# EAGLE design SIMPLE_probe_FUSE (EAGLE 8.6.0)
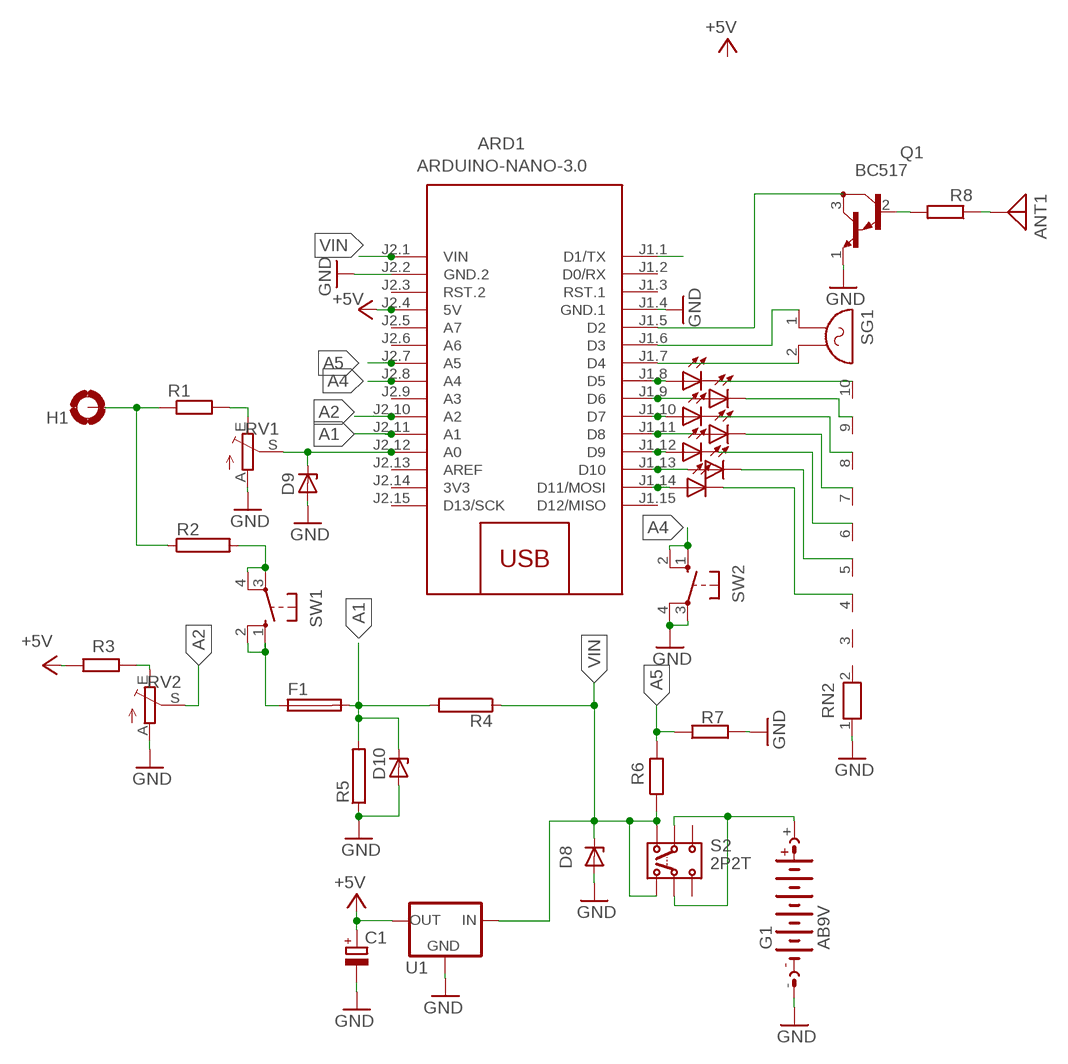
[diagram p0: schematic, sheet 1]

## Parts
ANT1  ANTENNA  [PAD-01]
ARD1  ARDUINO-NANO-3.0  [ARDUINO-NANO-3.0]
C1  CPOL-EUE2.5-6  [E2,5-6]
D1  LED5MM  [LED5MM]
D2  LED5MM  [LED5MM]
D3  LED5MM  [LED5MM]
D4  LED5MM  [LED5MM]
D5  LED5MM  [LED5MM]
D6  LED5MM  [LED5MM]
D7  LED5MM  [LED5MM]
D8  BZY97  [F126Z12]
D9  BZY97  [F126Z12]
D10  BZY97  [F126Z12]
F1  TE5  [TE5]
G1  AB9V  [AB9V]
H1  MOUNT-PAD-ROUND5.0  [5,0-PAD]
Q1  BC517  [TO92]
R1  R-EU_0617/22  [0617/22]
R2  RRWM4X22  [RWM4X22]
R3  R-EU_R1206  [R1206]
R4  RRWM4X22  [RWM4X22]
R5  RRWM4X22  [RWM4X22]
R6  R-EU_R1206  [R1206]
R7  R-EU_R1206  [R1206]
R8  R-EU_R1206  [R1206]
RN2  RN09  [RN-10]
RV1  TRIM_EU-CT6  [CT6]
RV2  TRIM_EU-CT6  [CT6]
S2  2P2T  [2P2T]
SG1  F/HGP  [F/HGP]
SW1  40-XX  [B3F-40XX]
SW2  40-XX  [B3F-40XX]
U1  78LXX  [78LXX]

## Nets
+5V: ARD1.J2.4(5V) C1.+ R3.1 U1.OUT
A1: ARD1.J2.11(A1) D10.C F1.2 R4.2 R5.2
A2: ARD1.J2.10(A2) RV2.S
A4: ARD1.J2.8(A4) SW2.1(S) SW2.2(S1)
A5: ARD1.J2.7(A5) R6.2 R7.1
GND: ARD1.J1.4(GND.1) ARD1.J2.2(GND.2) C1.- D8.A D9.A D10.A G1.- Q1.1(E) R5.1 R7.2 RN2.1 RV1.A RV2.A SW2.3(P) SW2.4(P1) U1.GND
N$1: ARD1.J1.1(D1/TX)
N$2: Q1.2(B) R8.2
N$3: ANT1.1 R8.1
N$4: R1.2 RV1.E
N$5: ARD1.J1.8(D5) D6.A
N$6: D6.K(C) RN2.10
N$7: ARD1.J1.9(D6) D3.A
N$8: D3.K(C) RN2.9
N$9: ARD1.J1.10(D7) D5.A
N$10: ARD1.J1.11(D8) D1.A
N$11: ARD1.J1.12(D9) D2.A
N$12: ARD1.J1.13(D10) D4.A
N$13: ARD1.J1.14(D11/MOSI) D7.A
N$14: D5.K(C) RN2.8
N$15: D1.K(C) RN2.7
N$16: D2.K(C) RN2.6
N$17: ARD1.J1.7(D4) SG1.2
N$18: ARD1.J1.6(D3) SG1.1
N$19: D4.K(C) RN2.5
N$20: D7.K(C) RN2.4
N$21: ARD1.J1.5(D2) Q1.3(C)
N$22: ARD1.J2.12(A0) D9.C RV1.S
N$24: F1.1 SW1.1(S) SW1.2(S1)
N$25: R3.2 RV2.E
N$26: R2.2 SW1.3(P) SW1.4(P1)
N$27: H1.B5(MOUNT) R1.1 R2.1
N$34: G1.+ S2.2.1 S2.2.2
VIN: ARD1.J2.1(VIN) D8.C R4.1 R6.1 S2.1.1 S2.1.2 U1.IN
Unconnected: ARD1.J1.2(D0/RX) ARD1.J1.3(RST.1) ARD1.J1.15(D12/MISO) ARD1.J2.3(RST.2) ARD1.J2.5(A7) ARD1.J2.6(A6) ARD1.J2.9(A3) ARD1.J2.13(AREF) ARD1.J2.15(D13/SCK) RN2.2 RN2.3 S2.3.1 S2.3.2

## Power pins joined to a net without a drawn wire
3V3: ARD1.J2.14(3V3)

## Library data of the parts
ANT1 = discrete:ANTENNA: Antenna
ARD1 = diy-modules:ARDUINO-NANO-3.0: Arduino Nano 3.0 and compatible devices More details available here: https://www.arduino.cc/en/Main/ArduinoBoardNano Click here to find device on ebay.com
C1 = rcl:CPOL-EU: POLARIZED CAPACITOR, European symbol
D1-D7 = led:LED: LED
D8-D10 = diode:BZY97: Z DIODE
F1 = fuse:TE5: FUSE; OC_FARNELL: unknown; OC_NEWARK: unknown
G1 = battery:AB9V: 9-V BATTERY CLIP
H1 = holes:MOUNT-PAD-ROUND: MOUNTING PAD, round
Q1 = transistor:BC517: NPN BIPOLAR DARLINGTON TRANSISTOR
R1 R3 R6-R8 = rcl:R-EU_: RESISTOR, European symbol
R2 R4 R5 = resistor-power:R: Power Resitor; OC_FARNELL: unknown; OC_NEWARK: unknown
RN2 = resistor-net:RN09: RESISTOR NETWORK; OC_FARNELL: unknown; OC_NEWARK: unknown
RV1 RV2 = pot:TRIM_EU-: POTENTIOMETER
S2 = switch:2P2T: SLIDE SWITCH 2P2T Part No. SS-22F05-G(A)4 Source: CANAL ELECTRONIC CO., LTD .. switsch.pdf
SG1 = buzzer:F/HGP: BUZZER; OC_FARNELL: unknown; OC_NEWARK: unknown
SW1 SW2 = switch-omron:40-XX: OMRON SWITCH; MF: OMRON COMPONENTS USA; MPN: B3F-4000; OC_FARNELL: 176434; OC_NEWARK: 36K3105
U1 = v-reg:78LXX: VOLTAGE REGULATOR

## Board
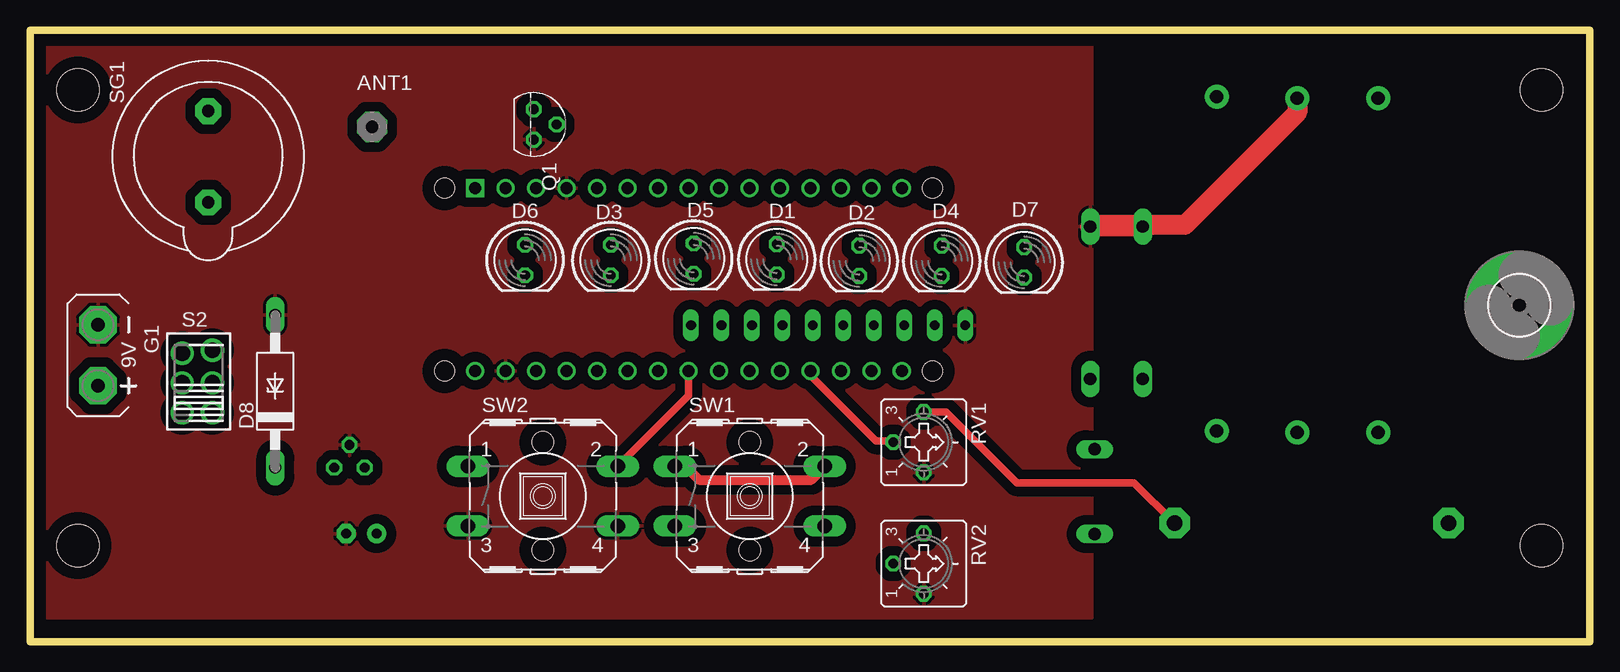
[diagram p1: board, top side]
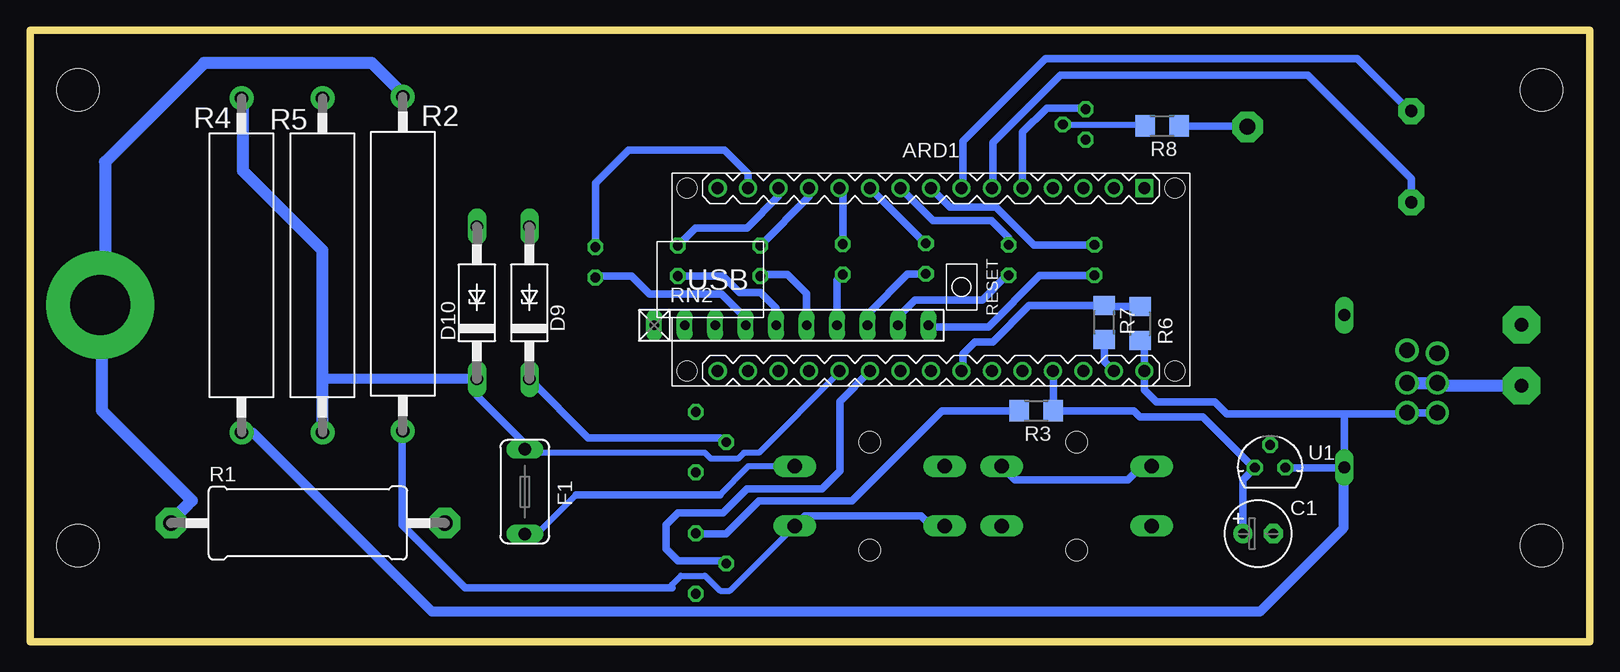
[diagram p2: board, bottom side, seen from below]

Size 130 x 51 mm. Coordinates in mm from the lower left corner, seen from the top.
Outline: 0,0 130,0 130,51 0,51 0,0
Copper layers (1*16): Top 0.035mm / dielectric 1.5mm / Bottom 0.035mm
Design rules "default": minimum track width 10mil, minimum drill 24mil, track to track 8mil, track to pad 8mil, pad to pad 8mil, via to via 8mil, smd to smd 8mil, copper to edge 40mil, drill to drill 8mil, minimum pad ring 10mil, minimum via ring 8mil, stop-mask expansion 4mil, vias tented up to drill 0mil, thermal gap 10mil
Holes 3.5 mm at 4,8 4,46 126,46 126,8

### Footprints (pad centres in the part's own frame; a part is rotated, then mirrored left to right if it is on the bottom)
PAD-01 = drill 1.321 pad 2.54 octagon: 1 0,0
ARDUINO-NANO-3.0 = drill 1 square: J1.1 17.78,7.62 | drill 1: J1.2 15.24,7.62; J1.3 12.7,7.62; J1.4 10.16,7.62; J1.5 7.62,7.62; J1.6 5.08,7.62; J1.7 2.54,7.62; J1.8 0,7.62; J1.9 -2.54,7.62; J1.10 -5.08,7.62; J1.11 -7.62,7.62; J1.12 -10.16,7.62; J1.13 -12.7,7.62; J1.14 -15.24,7.62; J1.15 -17.78,7.62; J2.1 17.78,-7.62; J2.2 15.24,-7.62; J2.3 12.7,-7.62; J2.4 10.16,-7.62; J2.5 7.62,-7.62; J2.6 5.08,-7.62; J2.7 2.54,-7.62; J2.8 0,-7.62; J2.9 -2.54,-7.62; J2.10 -5.08,-7.62; J2.11 -7.62,-7.62; J2.12 -10.16,-7.62; J2.13 -12.7,-7.62; J2.14 -15.24,-7.62; J2.15 -17.78,-7.62 | hole 1.651: -20.32,7.62; -20.32,-7.62; 20.32,-7.62; 20.32,7.62
E2,5-6 = drill 0.813 pad 1.6: + -1.27,0 | drill 0.813 pad 1.6 octagon: - 1.27,0
LED5MM = drill 0.813 octagon: A -1.27,0; K 1.27,0
F126Z12 = drill 1.016 long: A 6.35,0; C -6.35,0
TE5 = drill 1.016 long: 1 -3.54,0; 2 3.54,0
AB9V = drill 1.118 pad 3.15 octagon: + 0,2.54; - 0,-2.54
5,0-PAD = drill 5 pad 9: B5 0,0
TO92 = drill 0.813 octagon: 1 1.27,0; 2 0,1.905; 3 -1.27,0
0617/22 = drill 1.3 pad 2.54 octagon: 1 -11.43,0; 2 11.43,0
RWM4X22 = drill 1.1 pad 2: 1 -13.94,0; 2 13.94,0
R1206 = smd 1.6 x 1.803: 1 -1.422,0; 2 1.422,0
RN-10 = drill 0.813 long: 1 -11.43,0; 2 -8.89,0; 3 -6.35,0; 4 -3.81,0; 5 -1.27,0; 6 1.27,0; 7 3.81,0; 8 6.35,0; 9 8.89,0; 10 11.43,0
CT6 = drill 0.813 octagon: A 2.515,0; E -2.515,0; S 0,-2.54
2P2T = drill 1.3 pad 1.93: 1.1 -2.492,1.38; 1.2 -2.492,-1.126; 2.1 0,1.38; 2.2 0,-1.126; 3.1 2.492,1.38; 3.2 2.746,-1.126
F/HGP = drill 1.016 pad 2.159 octagon: 1 -3.81,0; 2 3.81,0
B3F-40XX = drill 1.194 long: 1 -6.248,2.489; 2 6.248,2.489; 3 -6.248,-2.489; 4 6.248,-2.489 | hole 1.803: 0,-4.496; 0,4.496
78LXX = drill 0.813 octagon: GND 0,1.905; IN 1.27,0; OUT -1.27,0

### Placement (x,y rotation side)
ANT1  28.52,42.94 0 top
ARD1  54.89,30.19 0 bottom
C1  27.62,9 0 bottom
D1  62.25,31.88 270 top
D2  69.12,31.75 270 top
D3  48.42,31.81 270 top
D4  76,31.75 270 top
D5  55.33,31.93 270 top
D6  41.27,31.81 270 top
D7  82.88,31.62 270 top
D8  20.44,20.87 90 top
D9  88.38,28.25 90 bottom
D10  92.75,28.25 90 bottom
F1  88.75,12.5 90 bottom
G1  5.67,23.87 180 top
H1  124.16,28.05 0 top
Q1  42,43.12 270 top
R1  106.83,9.88 0 bottom
R2  98.92,31.5 270 bottom
R3  46.12,19.25 180 bottom
R4  112.38,31.38 90 bottom
R5  105.62,31.38 270 bottom
R6  37.47,26.52 90 bottom
R7  40.45,26.61 270 bottom
R8  35.62,43 180 bottom
RN2  66.53,26.37 0 bottom
RV1  74.5,16.62 270 top
RV2  74.5,6.5 270 top
S2  14.07,21.56 90 top
SG1  14.85,40.44 90 top
SW1  60,12.12 0 top
SW2  42.75,12.12 0 top
U1  26.62,14.5 0 bottom

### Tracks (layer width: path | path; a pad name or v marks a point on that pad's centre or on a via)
+5V
  Bottom 0.61: ARD1.J2.4 44.7,22.54 R3.1 38,19.25 37.5,18.75 32.25,18.75 28,14.5 U1.OUT 28.89,13.5 C1.+
A1
  Bottom 0.5: ARD1.J2.11 62.51,22.49 69.25,15.75 70.5,15.75 71,15.25 73.25,15.25 73.75,15.75 88.46,15.75 F1.2
  Bottom 0.61: F1.2 88.75,16.5 92.75,20.5 D10.C
  Bottom 0.813: D10.C 105.53,21.9 105.62,22
  Bottom 1.016: R5.2 105.62,22 105.62,32.62 112.25,39.25 112.25,45.19 R4.2
A2
  Bottom 0.61: RV2.S 72.21,6.75 76,6.75 77,7.75 77,9.75 76,10.75 72.25,10.75 70.25,12.75 64,12.75 62.5,14.25 62.5,20.04 ARD1.J2.10
A4
  Top 0.61: ARD1.J2.8 54.89,20.51 SW2.2
  Bottom 0.61: SW2.1 37.39,14.61 38.5,13.5 47.88,13.5 SW2.2
A5
  Bottom 0.61: R6.2 40.37,27.94 R7.1 46.72,28.03 49.75,25 51.25,25 52.25,24 52.25,22.67 ARD1.J2.7
GND
  Top 1.676: D10.A 89,34.6 | 89,34.6 D9.A | R5.1 105.62,44.12 96.25,34.75 89.15,34.75 89,34.6
  Bottom 0.61: R7.2 40.45,23.37 ARD1.J2.2
  pour Top (isolate 0.813): 1,50 88.5,50 88.5,2 1,2
N$2
  Bottom 0.5: Q1.2 37.17,43.12 R8.2
N$3
  Bottom 0.61: R8.1 28.59,43 ANT1.1
N$4
  Top 0.61: RV1.E 76.36,19.14 82.25,13.25 92.04,13.25 R1.2
N$5
  Bottom 0.61: D6.A 46.33,33.08 49.5,36.25 53.33,36.25 ARD1.J1.8
N$6
  Bottom 0.61: D6.K 45.84,30.54 50.12,26.25 54.98,26.25 RN2.10
N$7
  Bottom 0.61: D3.A 48.42,33.67 49.88,35.12 54.74,35.12 ARD1.J1.9
N$8
  Bottom 0.61: D3.K 48.59,30.54 50.62,28.5 56.25,28.5 57.75,27 57.75,26.48 RN2.9
N$9
  Bottom 0.61: D5.A 55.37,33.2 ARD1.J1.10
N$10
  Bottom 0.61: D1.A 62.25,37.55 ARD1.J1.11
N$11
  Bottom 0.61: ARD1.J1.12 65.05,37.09 D2.A
N$12
  Bottom 0.61: ARD1.J1.13 67.59,37.16 70.25,34.5 74.52,34.5 D4.A
N$13
  Bottom 0.61: ARD1.J1.14 70.13,39.01 72.12,41 80.12,41 82.88,38.25 D7.A
N$14
  Bottom 0.61: D5.K 56.84,30.66 60.12,27.38 60.12,26.43 RN2.8
N$15
  Bottom 0.61: RN2.7 62.72,30.14 D1.K
N$16
  Bottom 0.61: RN2.6 65.26,29.01 66.88,30.62 68.98,30.62 D2.K
N$17
  Bottom 0.61: SG1.2 14.99,44.24 19.38,48.62 45.38,48.62 52.25,41.75 52.25,37.91 ARD1.J1.7
N$18
  Bottom 0.61: SG1.1 14.85,38.6 23.5,47.25 44.12,47.25 49.75,41.62 49.75,37.87 ARD1.J1.6
N$19
  Bottom 0.61: RN2.5 67.8,27.8 69.12,29.12 70.88,29.12 72.25,30.5 75.98,30.5 D4.K
N$20
  Bottom 0.61: RN2.4 70.34,26.96 72.38,29 78.38,29 79.88,30.5 82.73,30.5 D7.K
N$21
  Bottom 0.61: ARD1.J1.5 47.27,42.48 45.25,44.5 42.1,44.5 Q1.3
N$22
  Top 0.61: ARD1.J2.12 65.05,22.2 70.5,16.75 71.83,16.75 RV1.S
  Bottom 0.61: RV1.S 72.12,16.62 72.5,17 83.47,17 D9.C
N$24
  Top 0.813: SW1.1 54.64,14.61 55.75,13.5 65.13,13.5 SW1.2
  Bottom 0.5: SW1.2 70.14,14.61 72.5,12.25 | 84.5,12.25 87.75,9 88.71,9 F1.1
  Bottom 0.61: 72.5,12.25 84.5,12.25
N$25
  Bottom 0.61: R3.2 54,19.25 61.5,11.75 69.25,11.75 72,9 74.48,9 RV2.E
N$26
  Bottom 0.5: 76.5,4.5 76.5,4.75 75.75,5.5 73.75,5.5 72.5,4.25 71.63,4.25 SW1.4
  Bottom 0.61: SW1.3 54.89,9.64 55.75,10.5 65.38,10.5 SW1.4 | 76.5,4.5 93.75,4.5 99,9.75 99,17.48 R2.2
N$27
  Bottom 1.016: R1.1 116.52,11.77 124,19.25 124,27.89 H1.B5 123.75,28.45 123.75,40 115.5,48.25 101.5,48.25 98.92,45.67 R2.1
N$34
  Bottom 1.016: G1.+ 12.46,21.33 S2.2.1 S2.2.2
VIN
  Bottom 0.61: R6.1 37.11,24.74 ARD1.J2.1 37.12,22.55 37.12,21 36.12,20 31.25,20 30.25,19 20.25,19 | U1.IN 20.46,14.5 D8.C 20.44,18.81 20.25,19 | S2.1.1 S2.1.2 15.26,19 20.25,19
  Bottom 0.813: D8.C 20.5,14.46 20.5,9.5 27.5,2.5 96.5,2.5 111.44,17.44 R4.1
